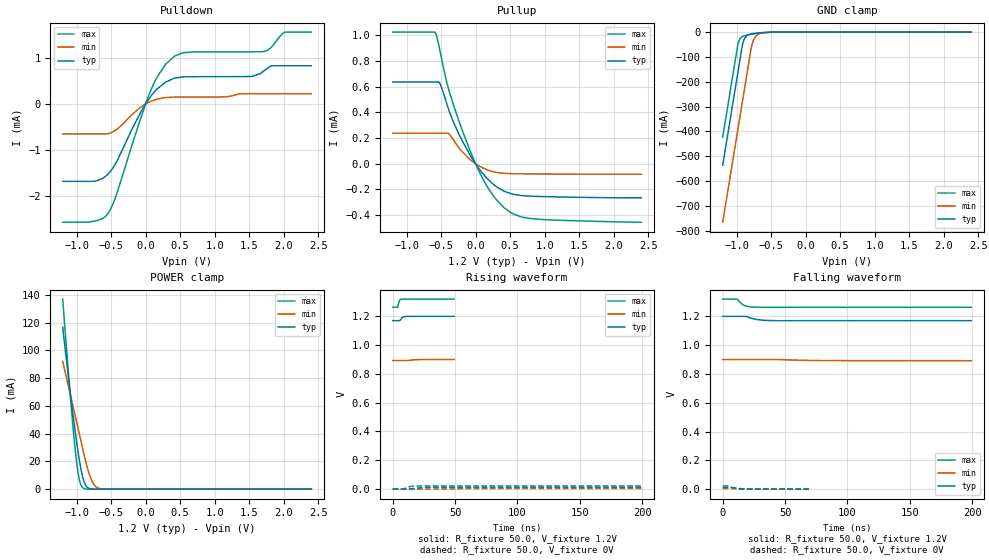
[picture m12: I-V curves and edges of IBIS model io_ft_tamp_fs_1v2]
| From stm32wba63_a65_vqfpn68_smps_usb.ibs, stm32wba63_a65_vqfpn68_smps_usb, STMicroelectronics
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[Model]   io_ft_tamp_fs_1v2
Model_type I/O
Polarity   Non-Inverting
Enable   Active-Low
| CAP_THRESHOLD on pad IOFT is "UDTCAPC" :
| Rising=30.0% of vddios   Falling=70.0% of vddios
| C_comp min and max val. don't necessarily correlate with the min and max pvt
| but are the smallest and greatest pad capacitance found.
| var   typ   min   max
C_comp   2.32869pF  2.27598pF  2.39710pF
|C_comp_pullup   1.36502pF  1.26597pF  1.45243pF
|C_comp_pulldown   963.66384fF  1.01002pF  944.67420fF
Vinl = 450.0mV
Vinh = 660.0mV
Vmeas = 600.0mV   | Reference voltage for timing measurements
Cref  = 50.0pF   | Timing specification test load capacitance value
Rref  = 1.0MOhm   | Timing specification test load resistance value
Vref  = 660.0mV   | Timing specification test load voltage
[Model Spec]
| TIME_THRESHOLD on pin ZIV11 is "CMOS" :
| Rising=50.0% of vdd   Falling=50.0% of vdd
Vinl 441.50000mV 335.50000mV 487.50000mV
Vinh 755.50000mV 552.50000mV 839.50000mV
| variable   typ   min   max
[Temperature Range] 25.0 140.0 -40.0
| variable   typ   min   max
[Voltage Range] 1.2V 900.0mV 1.32V
| variable   typ   min   max
[POWER Clamp Reference] 1.2V 900.0mV 1.32V
| variable   typ   min   max
[GND Clamp Reference] 0V 0V 0V
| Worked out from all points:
|   slope of the pulldown table from 0 to 0.18 V, typ, clamps not added: 522 ohm
|   slope of the pullup table from 0 to 0.18 V, typ, clamps not added: 1.49 kohm
|   GND clamp passes 1 mA (typ) near -0.54 V on its own axis
|   POWER clamp passes 1 mA (typ) near -0.83 V on its own axis
[POWER Clamp]
-1.2V     116.7mA    92.13mA    136.9mA
-1.09V    69.42mA    68.21mA    67.14mA
-1.02V    41.75mA    52.99mA    28.91mA
-990mV    30.98mA    46.47mA    16.09mA
-970mV    24.36mA    42.12mA    9.575mA
-940mV    15.59mA    35.6mA     3.485mA
-910mV    8.693mA    29.07mA    1.01mA
-860mV    2.259mA    18.59mA    104.6uA
-780mV    143.1uA    6.246mA    2.554uA
-720mV    16.22uA    1.846mA    157.1nA
-650mV    1.266uA    330.3uA    6.104nA
2.4V      0A         0A         0A
[GND Clamp]
-1.2V     -535.9mA   -765.1mA   -422.7mA
-990mV    -178.9mA   -408.1mA   -65.72mA
-970mV    -144.9mA   -374.1mA   -40.58mA
-920mV    -59.91mA   -289.1mA   -18.78mA
-900mV    -37.04mA   -255.1mA   -15.98mA
-880mV    -24.11mA   -221.1mA   -14.15mA
-780mV    -7.189mA   -55.54mA   -8.417mA
-750mV    -5.884mA   -29.71mA   -7.031mA
-700mV    -4.228mA   -11.41mA   -4.967mA
-610mV    -2.056mA   -3.105mA   -2.146mA
-390mV    -47.28uA   -188.8uA   -17.26uA
2.4V      740.6pA    197.9nA    245.1pA
| variable   typ   min   max
[Pullup Reference] 1.2V 900.0mV 1.32V
| variable   typ   min   max
[Pulldown Reference] 0V 0V 0V
[Pullup]
-1.2V     636.9uA    237.8uA    1.025mA
-580mV    636.9uA    237.8uA    1.017mA
-510mV    618.2uA    237.8uA    865.7uA
-440mV    507.1uA    237.8uA    686.1uA
-380mV    407.6uA    229.9uA    561.8uA
-250mV    241.3uA    130.7uA    346.6uA
-80mV     68.07uA    32.58uA    101.5uA
170mV     -115.1uA   -47.4uA    -178.3uA
420mV     -215.5uA   -74.74uA   -346.1uA
540mV     -237.3uA   -77.13uA   -389.8uA
790mV     -251.9uA   -78.78uA   -426uA
2.4V      -265.6uA   -81.56uA   -454.9uA
[Pulldown]
-1.2V     -1.691mA   -654.5uA   -2.583mA
-750mV    -1.69mA    -654.5uA   -2.563mA
-540mV    -1.526mA   -648.1uA   -2.381mA
-420mV    -1.264mA   -558.3uA   -1.971mA
-80mV     -206.7uA   -79.1uA    -354.6uA
80mV      176uA      59.82uA    314uA
290mV     478.8uA    141.1uA    868.7uA
420mV     565.7uA    150.4uA    1.047mA
1.54V     603uA      226.8uA    1.14mA
1.72V     729uA      226.8uA    1.15mA
2.01V     836.2uA    226.8uA    1.564mA
2.4V      836.2uA    226.8uA    1.572mA
[Ramp]
dV/dt_r 7.74265mV/8.00643ns 2.37319mV/21.38956ns 13.24855mV/4.61175ns
dV/dt_f 17.94413mV/8.48771ns 4.53508mV/21.30866ns 34.19538mV/5.22482ns
R_load = 50.0
| Removed startup time: 0s 0s 0s  .
| Removed end time: 49.25ns.
[Rising Waveform]
R_fixture   = 50.0
V_fixture   = 1.2V
V_fixture_min = 900.0mV
V_fixture_max = 1.32V
0s        1.17V      892.4mV    1.263V
3.85ns    1.17V      892.4mV    1.263V
5ns       1.17V      892.4mV    1.299V
5.45ns    1.17V      892.4mV    1.309V
6.15ns    1.175V     892.4mV    1.317V
7.05ns    1.186V     892.4mV    1.319V
8.35ns    1.196V     892.4mV    1.319V
11.05ns   1.2V       892.4mV    1.32V
21.15ns   1.2V       899.3mV    1.32V
49.25ns   1.2V       900mV      1.32V
| Removed startup time: 0s 0s 0s  .
| Removed end time: 199.25ns.
[Falling Waveform]
R_fixture   = 50.0
V_fixture   = 1.2V
V_fixture_min = 900.0mV
V_fixture_max = 1.32V
0s        1.2V       900mV      1.32V
11.75ns   1.2V       900mV      1.319V
14.8ns    1.2V       900mV      1.29V
17.35ns   1.2V       900mV      1.276V
19.3ns    1.199V     900mV      1.27V
20.7ns    1.193V     900mV      1.268V
27.6ns    1.178V     900mV      1.264V
44.75ns   1.17V      899.9mV    1.263V
85.4ns    1.17V      892.9mV    1.263V
199.3ns   1.17V      892.4mV    1.263V
| Removed startup time: 0s 0s 0s  .
| Removed end time: 199.25ns.
[Rising Waveform]
R_fixture   = 50.0
V_fixture   = 0V
V_fixture_min = 0V
V_fixture_max = 0V
0s        10.49nV    318.6nV    9.881nV
8.4ns     -368.2uV   1.435uV    -112.6uV
12.4ns    -74.94uV   -51.63uV   13.05mV
14.7ns    973.1uV    -99uV      18.12mV
17.85ns   4.733mV    -95.1uV    20.97mV
22.05ns   8.994mV    -102.8uV   21.85mV
28.45ns   11.92mV    -35.08uV   22.05mV
40.65ns   12.83mV    377.2uV    22.07mV
77.3ns    12.9mV     3.668mV    22.08mV
199.3ns   12.9mV     3.956mV    22.08mV
| Removed startup time: 0s 0s 0s  .
| Removed end time: 69.2ns.
[Falling Waveform]
R_fixture   = 50.0
V_fixture   = 0V
V_fixture_min = 0V
V_fixture_max = 0V
0s        12.91mV    3.962mV    22.08mV
3.95ns    12.9mV     3.962mV    22.09mV
5.95ns    12.86mV    3.961mV    15.51mV
9.9ns     7.889mV    3.962mV    4.863mV
11.85ns   5.761mV    3.954mV    1.719mV
14.3ns    3.478mV    3.522mV    405.8uV
18.35ns   920.5uV    2.831mV    140.8uV
22.6ns    217.2uV    2.169mV    60.18uV
39.55ns   21.47uV    365uV      1.691uV
69.2ns    313.4nV    25.38uV    26.52nV
